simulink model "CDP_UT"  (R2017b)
settings: Solver=FixedStepDiscrete  StartTime=0.0  StopTime=10.0  FixedStep=0.01  RelTol=1e-3  EnableMultiTasking=on
undefined symbols (not defined in the file): ASWTYPE_FALSE, ASWTYPE_TRUE, CaCDP_CellTempNTCVoltTable_mV, CaCDP_CellTempTable_C, CaCDP_CMUPCBTempNTCVoltTable_mV, CaCDP_CMUPCBTempTable_C, CbCDP_DiffBusbarTempStateCheck_flg, CbCDP_DiffCellTempStateCheck_flg, CbCDP_DiffCellVoltStateCheck_flg, CbCDP_IgnorUpdateVld_flg, CbCDP_MaxBusbarTempStateCheck_flg, CbCDP_MaxCellTempStateCheck_flg, CbCDP_MaxCellVoltStateCheck_flg, CbCDP_MinBusbarTempStateCheck_flg, CbCDP_MinCellTempStateCheck_flg, CbCDP_MinCellVoltStateCheck_flg, CcCDP_AFETempConfig_numb, CcCDP_AFETempFltThd_C, CcCDP_AFETempFltThdHys_C, CcCDP_BusbarTempRngFltHiThrd_C, CcCDP_BusbarTempRngFltLowThrd_C, CcCDP_CellDiffFltLevel1_mV, CcCDP_CellDiffFltLevel2_mV, CcCDP_CellDiffFltLevel3_mV, CcCDP_CellTempLowerLimit_C, CcCDP_CellTempRngFltHiThrd_C, CcCDP_CellTempRngFltLowThrd_C, CcCDP_CellTempUpperLimit_C, CcCDP_CellVoltConfig_numb, CcCDP_CellVoltLowerLimit_mV, CcCDP_CellVoltRngHiThrd_mV, CcCDP_CellVoltRngLowThrd_mV, CcCDP_CellVoltUpdateThrd_numb, CcCDP_CellVoltUpperLimit_mV, CcCDP_ChrgMaxCellTempFltLv1Thrd_C, CcCDP_ChrgMaxCellTempFltLv2Thrd_C, CcCDP_ChrgMaxCellTempFltLv3Thrd_C, CcCDP_ChrgMaxCellTempReturnDiff_C, CcCDP_ChrgMinCellTempFltLv1Thrd_C, CcCDP_ChrgMinCellTempFltLv2Thrd_C, CcCDP_ChrgMinCellTempFltLv3Thrd_C, CcCDP_ChrgMinCellTempReturnDiff_C, CcCDP_CMUPCBTempConfig_numb, CcCDP_CMUPCBTempFltThd_C, CcCDP_CMUPCBTempFltThdHys_C, CcCDP_DiffBusbarTempFltLevel1Thrd_C, CcCDP_DiffBusbarTempFltLevel2Thrd_C, CcCDP_DiffBusbarTempReturnDifference_C, CcCDP_DiffCellTempFltLevel1Thrd_C, CcCDP_DiffCellTempFltLevel2Thrd_C, CcCDP_DiffCellTempReturnDifference_C, CcCDP_DiffCellVoltReturnDifference_mV, CcCDP_DiffVoltCheckMaxCellTempCondition_C, CcCDP_DiffVoltCheckMaxCellVoltCondition_mV, CcCDP_DiffVoltCheckMinCellTempCondition_C, CcCDP_DiffVoltCheckMinCellVoltCondition_mV, CcCDP_DiffVoltCheckPackCurrCondition_A, CcCDP_MaxAFETempIniVal_C, CcCDP_MaxBusbarTempFltLevel1Thrd_C, CcCDP_MaxBusbarTempFltLevel2Thrd_C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
libraries: AIWAYS_Powertrain_BMS_lib x148, simulink x8
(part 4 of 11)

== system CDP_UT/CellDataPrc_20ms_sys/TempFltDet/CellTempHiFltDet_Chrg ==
  GbCDP_AllCellTempVld_flg : Inport
  GcCDP_MaxCellTemp_C : Inport  Port=2
  LbCDP_AnyCellTempVld_flg : Inport  Port=3
  LbCDP_ChrgWkUp_flg : Inport  Port=4
  ChrgCellTempHiFltDet_sys : Subsystem
  ChrgMaxTempCheck_Condition : Subsystem
  GbCDP_ChrgCellTempHiFltLv3_flg : Outport
  GbCDP_ChrgCellTempHiFltLv2_flg : Outport  Port=2
  GbCDP_ChrgCellTempHiFltLv1_flg : Outport  Port=3
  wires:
  LbCDP_ChrgWkUp_flg/1 -> ChrgMaxTempCheck_Condition/3(LbCDP_ChrgWkUp_flg)
  ChrgMaxTempCheck_Condition/1(LbCDP_ChrgMaxTempChkCond_flg) -> ChrgCellTempHiFltDet_sys/1(LbCDP_ChrgMaxTempChkCond_flg)
  LbCDP_AnyCellTempVld_flg/1 -> ChrgMaxTempCheck_Condition/2(LbCDP_AnyCellTempVld_flg)
  ChrgCellTempHiFltDet_sys/3(GbCDP_ChrgCellTempHiFltLv1_flg) -> GbCDP_ChrgCellTempHiFltLv1_flg/1
  ChrgCellTempHiFltDet_sys/2(GbCDP_ChrgCellTempHiFltLv2_flg) -> GbCDP_ChrgCellTempHiFltLv2_flg/1
  ChrgCellTempHiFltDet_sys/1(GbCDP_ChrgCellTempHiFltLv3_flg) -> GbCDP_ChrgCellTempHiFltLv3_flg/1
  GbCDP_AllCellTempVld_flg/1 -> ChrgMaxTempCheck_Condition/1(GbCDP_AllCellTempVld_flg)
  GcCDP_MaxCellTemp_C/1 -> ChrgCellTempHiFltDet_sys/2(GcCDP_MaxCellTemp_C)

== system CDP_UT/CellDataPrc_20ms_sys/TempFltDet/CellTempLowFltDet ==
  GbCDP_AllCellTempVld_flg : Inport
  GcCDP_MinCellTemp_C : Inport  Port=2
  LbCDP_AnyCellTempVld_flg : Inport  Port=3
  LbCDP_ChrgWkUp_flg : Inport  Port=4
  MinCellTemp_SateSwitch_Sys : Subsystem
  MinTempCheck_Condition : Subsystem
  GbCDP_CellTempLowFltLv3_flg : Outport
  GbCDP_CellTempLowFltLv2_flg : Outport  Port=2
  GbCDP_CellTempLowFltLv1_flg : Outport  Port=3
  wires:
  GcCDP_MinCellTemp_C/1 -> MinCellTemp_SateSwitch_Sys/2(GcCDP_MinCellTemp_C)
  GbCDP_AllCellTempVld_flg/1 -> MinTempCheck_Condition/1(GbCDP_AllCellTempVld_flg)
  MinCellTemp_SateSwitch_Sys/1(GbCDP_CellTempLowFltLv3_flg) -> GbCDP_CellTempLowFltLv3_flg/1
  MinCellTemp_SateSwitch_Sys/2(GbCDP_CellTempLowFltLv2_flg) -> GbCDP_CellTempLowFltLv2_flg/1
  MinCellTemp_SateSwitch_Sys/3(GbCDP_CellTempLowFltLv1_flg) -> GbCDP_CellTempLowFltLv1_flg/1
  LbCDP_AnyCellTempVld_flg/1 -> MinTempCheck_Condition/2(LbCDP_AnyCellTempVld_flg)
  MinTempCheck_Condition/1(LbCDP_MinTempCheckCondition_flg) -> MinCellTemp_SateSwitch_Sys/1(LbCDP_MinTempCheckCondition_flg)
  LbCDP_ChrgWkUp_flg/1 -> MinTempCheck_Condition/3(LbCDP_ChrgWkUp_flg)

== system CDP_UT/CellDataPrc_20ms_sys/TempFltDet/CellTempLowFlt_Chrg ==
  GbCDP_AllCellTempVld_flg : Inport
  GcCDP_MinCellTemp_C : Inport  Port=2
  LbCDP_AnyCellTempVld_flg : Inport  Port=3
  LbCDP_ChrgWkUp_flg : Inport  Port=4
  ChrgMinCellTemp_SateSwitch_Sys : Subsystem
  ChrgMinTempCheck_Condition : Subsystem
  GbCDP_ChrgCellTempLowFltLv3_flg : Outport
  GbCDP_ChrgCellTempLowFltLv2_flg : Outport  Port=2
  GbCDP_ChrgCellTempLowFltLv1_flg : Outport  Port=3
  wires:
  LbCDP_ChrgWkUp_flg/1 -> ChrgMinTempCheck_Condition/3(LbCDP_ChrgWkUp_flg)
  ChrgMinTempCheck_Condition/1(LbCDP_ChrgMinTempChkCond_flg) -> ChrgMinCellTemp_SateSwitch_Sys/1(LbCDP_ChrgMinTempChkCond_flg)
  LbCDP_AnyCellTempVld_flg/1 -> ChrgMinTempCheck_Condition/2(LbCDP_AnyCellTempVld_flg)
  ChrgMinCellTemp_SateSwitch_Sys/3(GbCDP_ChrgCellTempLowFltLv1_flg) -> GbCDP_ChrgCellTempLowFltLv1_flg/1
  ChrgMinCellTemp_SateSwitch_Sys/2(GbCDP_ChrgCellTempLowFltLv2_flg) -> GbCDP_ChrgCellTempLowFltLv2_flg/1
  ChrgMinCellTemp_SateSwitch_Sys/1(GbCDP_ChrgCellTempLowFltLv3_flg) -> GbCDP_ChrgCellTempLowFltLv3_flg/1
  GbCDP_AllCellTempVld_flg/1 -> ChrgMinTempCheck_Condition/1(GbCDP_AllCellTempVld_flg)
  GcCDP_MinCellTemp_C/1 -> ChrgMinCellTemp_SateSwitch_Sys/2(GcCDP_MinCellTemp_C)

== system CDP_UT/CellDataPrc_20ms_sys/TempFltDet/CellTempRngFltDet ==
  GcCDP_MaxCellTemp_C : Inport
  GcCDP_MinCellTemp_C : Inport  Port=2
  LbCDP_AnyCellTempVld_flg : Inport  Port=3
  CellTempRngHiFltDet_sys : Subsystem
  CellTempRngLowFltDet_sys : Subsystem
  TempRngHiCheck_Condition : Subsystem
  TempRngLowCheck_Condition : Subsystem
  GbCDP_CellTempRngHiFlt_flg : Outport
  GbCDP_CellTempRngLowFlt_flg : Outport  Port=2
  LbCDP_CellTempRngHiFlt_flg : Outport  Port=3
  LbCDP_CellTempRngLowFlt_flg : Outport  Port=4
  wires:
  GcCDP_MaxCellTemp_C/1 -> CellTempRngHiFltDet_sys/2(GcCDP_MaxCellTemp_C)
  LbCDP_AnyCellTempVld_flg/1 -> TempRngLowCheck_Condition/1(LbCDP_AnyCellTempVld_flg), TempRngHiCheck_Condition/1(LbCDP_AnyCellTempVld_flg)
  CellTempRngHiFltDet_sys/1(LbCDP_CellTempRngHiFlt_flg) -> LbCDP_CellTempRngHiFlt_flg/1
  CellTempRngHiFltDet_sys/2(GbCDP_CellTempRngHiFlt_flg) -> GbCDP_CellTempRngHiFlt_flg/1
  GcCDP_MinCellTemp_C/1 -> CellTempRngLowFltDet_sys/2(GcCDP_MinCellTemp_C)
  TempRngLowCheck_Condition/1(LbCDP_CellTempRngLowChk_flg) -> CellTempRngLowFltDet_sys/1(LbCDP_CellTempRngLowChk_flg)
  CellTempRngLowFltDet_sys/1(LbCDP_CellTempRngLowFlt_flg) -> LbCDP_CellTempRngLowFlt_flg/1
  CellTempRngLowFltDet_sys/2(GbCDP_CellTempRngLowFlt_flg) -> GbCDP_CellTempRngLowFlt_flg/1
  TempRngHiCheck_Condition/1(LbCDP_CellTempRngHiChk_flg) -> CellTempRngHiFltDet_sys/1(LbCDP_CellTempRngHiChk_flg)

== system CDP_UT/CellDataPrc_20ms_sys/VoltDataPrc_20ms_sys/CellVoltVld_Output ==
  GaISP_CellVoltVld_numb : Inport
  GeISP_CmuReIninSts_enum : Inport  Port=2
  Bitwise Logical Operator : simulink/Logic and Bit Operations/Bitwise Operator  logicop=AND  UseBitMask=on  BitMask=CDP_CONST97_NUMB  BitMaskRealWorld=Stored Integer
  Constant1 : Constant  Value=Enum_ISPCmuReIninSts.Enum_ISPCmuReIninSts_InintProcess
  Constant2 : Constant  Value=CDP_CONST0_NUMB
  Data Type Conversion : DataTypeConversion
  Logical Operator2 : Logic  Operator=OR  AllPortsSameDT=off  OutDataTypeStr=boolean
  OverWrite5 : AIWAYS_Powertrain_BMS_lib/Signals/OverWrite  OverWrite_Value=CaCDP_CellVoltVldOvr_flg  OverWrite_flag=CbCDP_CellVoltVldOvrSwt_flg
  Relational Operator1 : RelationalOperator  Operator===  OutDataTypeStr=boolean
  Relational Operator2 : RelationalOperator  Operator===  OutDataTypeStr=boolean
  LaCDP_CellVoltVld_flg : Outport
  GaCDP_CellVoltVld_flg : Outport  Port=2
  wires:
  OverWrite5/1 -> GaCDP_CellVoltVld_flg/1  "GaCDP_CellVoltVld_flg"
  GeISP_CmuReIninSts_enum/1 -> Data Type Conversion/1
  Logical Operator2/1 -> LaCDP_CellVoltVld_flg/1, OverWrite5/1  "LaCDP_CellVoltVld_flg"
  Relational Operator1/1 -> Logical Operator2/2
  Constant1/1 -> Relational Operator1/2
  Data Type Conversion/1 -> Relational Operator1/1
  Relational Operator2/1 -> Logical Operator2/1
  Constant2/1 -> Relational Operator2/2
  GaISP_CellVoltVld_numb/1 -> Bitwise Logical Operator/1
  Bitwise Logical Operator/1 -> Relational Operator2/1

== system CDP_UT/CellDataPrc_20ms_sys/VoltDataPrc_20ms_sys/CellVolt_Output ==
  GaISP_CellVolt_mV : Inport
  GaISP_CellVoltVld_numb : Inport  Port=2
  GeISP_CmuReIninSts_enum : Inport  Port=3
  GaISP_CellVoltUpdCnt_numb : Inport  Port=4
  GeUDS_CapSel_enum : Inport  Port=5
  GcUDS_CellVoltNum_numb : Inport  Port=6
  Bitwise Logical Operator : simulink/Logic and Bit Operations/Bitwise Operator  logicop=AND  UseBitMask=on  BitMask=CDP_CONST97_NUMB  BitMaskRealWorld=Stored Integer
  CellVolt_SignalFilt : Subsystem
  Comparison1 : RelationalOperator  Operator===  OutDataTypeStr=boolean
  Comparison4 : RelationalOperator  Operator===  OutDataTypeStr=boolean
  Constant1 : Constant  Value=Enum_ISPCmuReIninSts.Enum_ISPCmuReIninSts_InintProcess
  Constant2 : Constant  Value=CDP_CONST0_NUMB
  Constant3 : Constant  Value=CDP_CONST0_NUMB
  Constant4 : Constant  Value=CbCDP_IgnorUpdateVld_flg
  Constant5 : Constant  Value=ASWTYPE_FALSE
  Data Type Conversion : DataTypeConversion
  Logical Operator1 : Logic  Operator=OR  AllPortsSameDT=off  OutDataTypeStr=boolean
  Logical Operator2 : Logic  Operator=OR  AllPortsSameDT=off  OutDataTypeStr=boolean
  Relational Operator : RelationalOperator  Operator=~=  OutDataTypeStr=boolean
  Relational Operator1 : RelationalOperator  Operator===  OutDataTypeStr=boolean
  Switch : Switch  Criteria=u2 ~= 0
  Switch1 : Switch  Criteria=u2 ~= 0  Threshold=1  RndMeth=Zero
  Unit Delay : UnitDelay  SampleTime=-1  StateName=StateName
  LaCDP_CellVolt_mV : Outport
  GaCDP_CellVolt_mV : Outport  Port=2
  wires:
  Data Type Conversion/1 -> Relational Operator1/1
  Switch/1 -> CellVolt_SignalFilt/1(LaCDP_CellVolt_mV), LaCDP_CellVolt_mV/1, Unit Delay/1  "LaCDP_CellVolt_mV"
  Constant1/1 -> Relational Operator1/2
  Relational Operator1/1 -> Logical Operator2/2
  GaISP_CellVoltVld_numb/1 -> Bitwise Logical Operator/1
  GaISP_CellVolt_mV/1 -> Switch/3
  Logical Operator2/1 -> CellVolt_SignalFilt/2(LaCDP_CellVoltUpdateVld_flg), Switch/2
  Unit Delay/1 -> Switch/1
  GeISP_CmuReIninSts_enum/1 -> Data Type Conversion/1
  Constant2/1 -> Relational Operator/2
  Bitwise Logical Operator/1 -> Relational Operator/1
  Relational Operator/1 -> Logical Operator1/1, Switch1/1
  GaISP_CellVoltUpdCnt_numb/1 -> Comparison4/1
  Constant4/1 -> Switch1/2
  Constant3/1 -> Comparison4/2
  Logical Operator1/1 -> Switch1/3
  Comparison4/1 -> Comparison1/1
  Switch1/1 -> Logical Operator2/1
  Constant5/1 -> Comparison1/2
  Comparison1/1 -> Logical Operator1/2
  GeUDS_CapSel_enum/1 -> CellVolt_SignalFilt/3(GeUDS_CapSel_enum)
  CellVolt_SignalFilt/1(GaCDP_CellVolt_mV) -> GaCDP_CellVolt_mV/1
  GcUDS_CellVoltNum_numb/1 -> CellVolt_SignalFilt/4(GcUDS_CellVoltNum_numb)

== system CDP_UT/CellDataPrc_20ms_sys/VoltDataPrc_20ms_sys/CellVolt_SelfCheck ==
  GeMSM_BMUState_enum : Inport
  GbCDP_SumCellVoltVld_flg : Inport  Port=2
  GcCDP_MaxCellVolt_mV : Inport  Port=3
  GcCDP_MinCellVolt_mV : Inport  Port=4
  Constant : Constant  Value=Enum_MSMBMUState.Enum_MSMBMUState_Standby
  Constant1 : Constant  Value=ASWTYPE_TRUE
  Constant2 : Constant  Value=CcCDP_CellVoltLowerLimit_mV
  Constant3 : Constant  Value=CcCDP_CellVoltUpperLimit_mV
  Data Type Conversion1 : DataTypeConversion
  Logical Operator : Logic  Inputs=4  AllPortsSameDT=off  OutDataTypeStr=boolean
  OverWrite : AIWAYS_Powertrain_BMS_lib/Signals/OverWrite  OverWrite_Value=CbCDP_CellVoltSelfChckOvr_flg  OverWrite_flag=CbCDP_CellVoltSelfChckOvrSwt_flg
  Relational Operator : RelationalOperator  Operator===  OutDataTypeStr=boolean
  Relational Operator1 : RelationalOperator  OutDataTypeStr=boolean
  Relational Operator2 : RelationalOperator  Operator=<=  OutDataTypeStr=boolean
  Relational Operator4 : RelationalOperator  Operator===  OutDataTypeStr=boolean
  GbCDP_CellVoltSelfChck_flg : Outport
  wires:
  GeMSM_BMUState_enum/1 -> Data Type Conversion1/1
  Constant/1 -> Relational Operator4/2
  Relational Operator1/1 -> Logical Operator/3
  Relational Operator2/1 -> Logical Operator/2
  Logical Operator/1 -> OverWrite/1
  GcCDP_MinCellVolt_mV/1 -> Relational Operator1/1
  Constant2/1 -> Relational Operator1/2
  GbCDP_SumCellVoltVld_flg/1 -> Relational Operator/1
  Constant1/1 -> Relational Operator/2
  Relational Operator/1 -> Logical Operator/1
  OverWrite/1 -> GbCDP_CellVoltSelfChck_flg/1  "GbCDP_CellVoltSelfChck_flg"
  GcCDP_MaxCellVolt_mV/1 -> Relational Operator2/1
  Constant3/1 -> Relational Operator2/2
  Relational Operator4/1 -> Logical Operator/4
  Data Type Conversion1/1 -> Relational Operator4/1

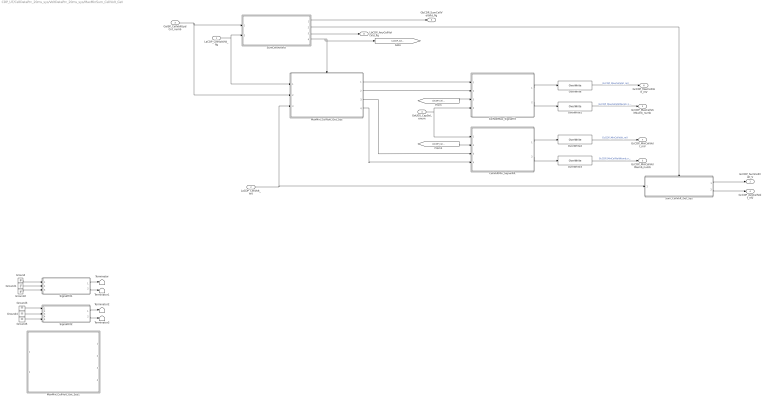
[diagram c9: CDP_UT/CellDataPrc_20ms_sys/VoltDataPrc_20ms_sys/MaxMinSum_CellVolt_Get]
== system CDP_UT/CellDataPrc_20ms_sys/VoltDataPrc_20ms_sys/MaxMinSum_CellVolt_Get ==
  LaCDP_CellVoltVld_flg : Inport
  LaCDP_CellVolt_mV : Inport  Port=2
  GaISP_CellVoltUpdCnt_numb : Inport  Port=3
  GeUDS_CapSel_enum : Inport  Port=4
  CellVoltMax_SignalFilt : Subsystem
  CellVoltMin_SignalFilt : Subsystem
  Ground{,1..5} (6 alike) : Ground
  MaxMin_CellVolt_Get_Sys : Subsystem
  MaxMin_CellVolt_Get_Sys1 : Subsystem  Commented=on
  OverWrite : AIWAYS_Powertrain_BMS_lib/Signals/OverWrite  OverWrite_Value=CcCDP_MaxCellVoltOvr_mV  OverWrite_flag=CbCDP_MaxCellVoltOvrSwt_flg
  OverWrite1 : AIWAYS_Powertrain_BMS_lib/Signals/OverWrite  OverWrite_Value=CcCDP_MaxCellVoltNumbOvr_numb  OverWrite_flag=CbCDP_MaxCellVoltNumbOvrSwt_flg
  OverWrite2 : AIWAYS_Powertrain_BMS_lib/Signals/OverWrite  OverWrite_Value=CcCDP_MinCellVoltOvr_mV  OverWrite_flag=CbCDP_MinCellVoltOvrSwt_flg
  OverWrite3 : AIWAYS_Powertrain_BMS_lib/Signals/OverWrite  OverWrite_Value=CcCDP_MinCellVoltNumbOvr_numb  OverWrite_flag=CbCDP_MinCellVoltNumbOvrSwt_flg
  SignalFilt1 : Subsystem  Commented=on
  SignalFilt2 : Subsystem  Commented=on
  SumCellVoltVld : Subsystem
  Sum_CellVolt_Get_Sys : Subsystem
  Terminator{,1..3} (4 alike) : Terminator
  GcCDP_SumCellVolt_V : Outport
  GcCDP_MaxCellVoltNumb_numb : Outport  Port=2
  GcCDP_MinCellVoltNumb_numb : Outport  Port=3
  GcCDP_AvgCellVolt_mV : Outport  Port=4
  GbCDP_SumCellVoltVld_flg : Outport  Port=5
  GcCDP_MaxCellVolt_mV : Outport  Port=6
  GcCDP_MinCellVolt_mV : Outport  Port=7
  LbCDP_AnyCellVoltVld_flg : Outport  Port=8
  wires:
  SumCellVoltVld/1(GbCDP_SumCellVoltVld_flg) -> GbCDP_SumCellVoltVld_flg/1
  LaCDP_CellVoltVld_flg/1 -> SumCellVoltVld/2(LaCDP_CellVoltVld_flg), MaxMin_CellVolt_Get_Sys/1(LaCDP_CellVoltVld_flg)
  LaCDP_CellVolt_mV/1 -> Sum_CellVolt_Get_Sys/1(LaCDP_CellVolt_mV), MaxMin_CellVolt_Get_Sys/3(LaCDP_CellVolt_mV)
  Sum_CellVolt_Get_Sys/1(GcCDP_SumCellVolt_V) -> GcCDP_SumCellVolt_V/1
  Sum_CellVolt_Get_Sys/2(GcCDP_AvgCellVolt_mV) -> GcCDP_AvgCellVolt_mV/1
  SumCellVoltVld/3(LbCDP_AnyCellVoltVld_flg) -> LbCDP_AnyCellVoltVld_flg/1
  SumCellVoltVld/2(LbCDP_SumCellVoltVld_flg) -> Sum_CellVolt_Get_Sys/Enable
  SignalFilt1/1(Output_Value) -> Terminator/1
  SignalFilt1/2(Output_Numb) -> Terminator1/1
  Ground/1 -> SignalFilt1/1(Input_Value)
  Ground1/1 -> SignalFilt1/2(Input_Numb)
  Ground2/1 -> SignalFilt1/3(GeUDS_CapSel_enum)
  Ground5/1 -> SignalFilt2/5(InputValueUpdate)
  Ground4/1 -> SignalFilt2/3(GeUDS_CapSel_enum)
  Ground3/1 -> SignalFilt2/1(Input_Value)
  SignalFilt2/2(Output_Numb) -> Terminator3/1
  SignalFilt2/1(Output_Value) -> Terminator2/1
  MaxMin_CellVolt_Get_Sys/1(LcCDP_MaxCellVolt_mV) -> CellVoltMax_SignalFilt/1(LcCDP_MaxCellVolt_mV)
  MaxMin_CellVolt_Get_Sys/2(LcCDP_MaxCellVoltNumb_numb) -> CellVoltMax_SignalFilt/2(LcCDP_MaxCellVoltNumb_numb)
  GaISP_CellVoltUpdCnt_numb/1 -> MaxMin_CellVolt_Get_Sys/2(GaISP_CellVoltUpdCnt_numb), SumCellVoltVld/1(GaISP_CellVoltUpdCnt_numb)
  CellVoltMax_SignalFilt/1(GcCDP_MaxCellVolt_mV) -> OverWrite/1
  OverWrite/1 -> GcCDP_MaxCellVolt_mV/1  "GcCDP_MaxCellVolt_mV"
  CellVoltMax_SignalFilt/2(GcCDP_MaxCellVoltNumb_numb) -> OverWrite1/1
  OverWrite1/1 -> GcCDP_MaxCellVoltNumb_numb/1  "GcCDP_MaxCellVoltNumb_numb"
  MaxMin_CellVolt_Get_Sys/3(LcCDP_MinCellVolt_mV) -> CellVoltMin_SignalFilt/3(LcCDP_MinCellVolt_mV)
  MaxMin_CellVolt_Get_Sys/4(LcCDP_MinCellVoltNumb_numb) -> CellVoltMin_SignalFilt/4(LcCDP_MinCellVoltNumb_numb)
  OverWrite2/1 -> GcCDP_MinCellVolt_mV/1  "GcCDP_MinCellVolt_mV"
  CellVoltMin_SignalFilt/1(GcCDP_MinCellVolt_mV) -> OverWrite2/1
  CellVoltMin_SignalFilt/2(GcCDP_MinCellVoltNumb_numb) -> OverWrite3/1
  OverWrite3/1 -> GcCDP_MinCellVoltNumb_numb/1  "GcCDP_MinCellVoltNumb_numb"
  SumCellVoltVld/4(LbCDP_CellVoltUpdateVld_flg) -> MaxMin_CellVolt_Get_Sys/Enable, [LbCDP_CellVoltUpdateVld_flg]
  GeUDS_CapSel_enum/1 -> CellVoltMin_SignalFilt/1(GeUDS_CapSel_enum), CellVoltMax_SignalFilt/4(GeUDS_CapSel_enum)
  [LbCDP_CellVoltUpdateVld_flg] -> CellVoltMax_SignalFilt/3(LbCDP_CellVoltUpdateVld_flg)
  [LbCDP_CellVoltUpdateVld_flg] -> CellVoltMin_SignalFilt/2(LbCDP_CellVoltUpdateVld_flg)

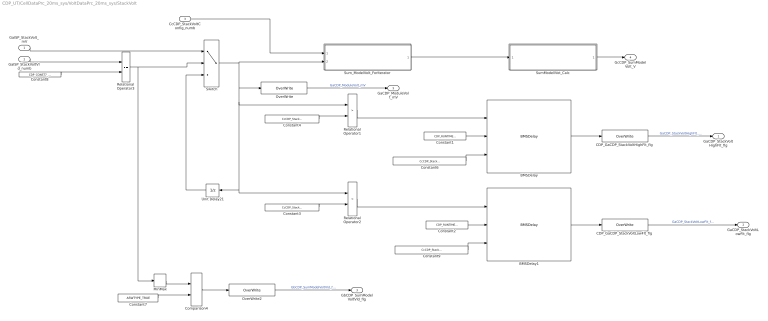
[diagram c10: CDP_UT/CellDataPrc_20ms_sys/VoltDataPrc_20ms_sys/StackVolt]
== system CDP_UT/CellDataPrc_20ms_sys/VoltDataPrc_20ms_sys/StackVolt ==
  GaISP_StackVolt_mV : Inport
  GaISP_StackVoltVld_numb : Inport  Port=2
  CcCDP_StackVoltConfig_numb : Inport  Port=3
  BMSDelay : AIWAYS_Powertrain_BMS_lib/Debounce & Delay/BMSDelay
  BMSDelay1 : AIWAYS_Powertrain_BMS_lib/Debounce & Delay/BMSDelay
  CDP_GaCDP_StackVoltHighFlt_flg : AIWAYS_Powertrain_BMS_lib/Signals/OverWrite  OverWrite_Value=CaCDP_StackVoltHighFltOvr_flg  OverWrite_flag=CbCDP_StackVoltHighFltOvrSwt_flg
  CDP_GaCDP_StackVoltLowFlt_flg : AIWAYS_Powertrain_BMS_lib/Signals/OverWrite  OverWrite_Value=CaCDP_StackVoltLowFltOvr_flg  OverWrite_flag=CbCDP_StackVoltLowFltOvrSwt_flg
  Comparison4 : RelationalOperator  Operator===  OutDataTypeStr=boolean
  Constant1 : Constant  Value=CDP_RUNTIME20_MS
  Constant2 : Constant  Value=CDP_RUNTIME20_MS
  Constant3 : Constant  Value=CcCDP_StackVoltLow_mV
  Constant4 : Constant  Value=CcCDP_StackVoltHigh_mV
  Constant6 : Constant  Value=CcCDP_StackVoltHighDelayTi_ms
  Constant7 : Constant  Value=ASWTYPE_TRUE
  Constant8 : Constant  Value=CDP_CONST7_NUMB
  Constant9 : Constant  Value=CcCDP_StackVoltLowDelayTi_ms
  MinMax : MinMax  OutDataTypeStr=Inherit: Inherit via back propagation  RndMeth=Zero
  OverWrite : AIWAYS_Powertrain_BMS_lib/Signals/OverWrite  OverWrite_Value=CaCDP_ModuleVoltOvr_mV  OverWrite_flag=CbCDP_ModuleVoltOvrSwt_flg
  OverWrite2 : AIWAYS_Powertrain_BMS_lib/Signals/OverWrite  OverWrite_Value=CbCDP_SumModelVoltVldOvr_flg  OverWrite_flag=CbCDP_SumModelVoltVldOvrSwt_flg
  Relational Operator1 : RelationalOperator  Operator=>  OutDataTypeStr=boolean
  Relational Operator2 : RelationalOperator  Operator=<  OutDataTypeStr=boolean
  Relational Operator3 : RelationalOperator  Operator===  OutDataTypeStr=boolean
  SumModellVot_Calc : Subsystem
  Sum_ModelVolt_ForIterator : Subsystem
  Switch : Switch  Criteria=u2 ~= 0  Threshold=1  RndMeth=Zero
  Unit Delay21 : UnitDelay  SampleTime=-1  StateName=StateName
  GaCDP_StackVoltHighFlt_flg : Outport
  GaCDP_StackVoltLowFlt_flg : Outport  Port=2
  GbCDP_SumModelVoltVld_flg : Outport  Port=3
  GcCDP_SumModelVolt_V : Outport  Port=4
  GaCDP_ModuleVolt_mV : Outport  Port=5
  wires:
  BMSDelay1/1 -> CDP_GaCDP_StackVoltLowFlt_flg/1
  CDP_GaCDP_StackVoltHighFlt_flg/1 -> GaCDP_StackVoltHighFlt_flg/1  "GaCDP_StackVoltHighFlt_flg"
  GaISP_StackVolt_mV/1 -> Switch/1
  CDP_GaCDP_StackVoltLowFlt_flg/1 -> GaCDP_StackVoltLowFlt_flg/1  "GaCDP_StackVoltLowFlt_flg"
  BMSDelay/1 -> CDP_GaCDP_StackVoltHighFlt_flg/1
  Relational Operator3/1 -> MinMax/1, Switch/2
  Unit Delay21/1 -> Switch/3
  Constant9/1 -> BMSDelay1/3
  Constant8/1 -> Relational Operator3/2
  Constant6/1 -> BMSDelay/3
  Relational Operator2/1 -> BMSDelay1/1
  Constant4/1 -> Relational Operator1/2
  Constant1/1 -> BMSDelay/2
  Relational Operator1/1 -> BMSDelay/1
  Constant3/1 -> Relational Operator2/2
  Constant2/1 -> BMSDelay1/2
  MinMax/1 -> Comparison4/1
  OverWrite2/1 -> GbCDP_SumModelVoltVld_flg/1  "GbCDP_SumModelVoltVld_flg"
  Constant7/1 -> Comparison4/2
  SumModellVot_Calc/1(GcCDP_SumModelVolt_V) -> GcCDP_SumModelVolt_V/1
  Comparison4/1 -> OverWrite2/1
  CcCDP_StackVoltConfig_numb/1 -> Sum_ModelVolt_ForIterator/1(CcCDP_StackVoltConfig_numb)
  Sum_ModelVolt_ForIterator/1(LcCDP_SumModelVolt_mV) -> SumModellVot_Calc/1(LcCDP_SumModelVolt_mV)
  GaISP_StackVoltVld_numb/1 -> Relational Operator3/1
  OverWrite/1 -> GaCDP_ModuleVolt_mV/1  "GaCDP_ModuleVolt_mV"
  Switch/1 -> OverWrite/1, Relational Operator2/1, Unit Delay21/1, Relational Operator1/1, Sum_ModelVolt_ForIterator/2(GaISP_StackVolt_mV)

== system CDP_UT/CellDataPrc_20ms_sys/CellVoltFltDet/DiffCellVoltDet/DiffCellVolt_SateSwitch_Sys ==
  LbCDP_DiffvoltCheckCondition_flg : Inport
  GcCDP_MaxCellVolt_mV : Inport  Port=2
  GcCDP_MinCellVolt_mV : Inport  Port=3
  LbCDP_CellVoltRngLowFlt_flg : Inport  Port=4
  LbCDP_CellVoltRngHiFlt_flg : Inport  Port=5
  Add : Sum  Inputs=+-
  Bus Creator : BusCreator  Inputs=4
  Bus Selector : BusSelector  OutputSignals=LcCDP_DiffCellVolt_mV,LbCDP_DiffvoltCheckCondition_flg,LbCDP_CellVoltRngLowFlt_flg,LbCDP_CellVoltRngHiFlt_flg
  Bus Selector1 : BusSelector  OutputSignals=LcCDP_DiffCellVolt_mV,LbCDP_DiffvoltCheckCondition_flg,LbCDP_CellVoltRngLowFlt_flg,LbCDP_CellVoltRngHiFlt_flg
  Bus Selector2 : BusSelector  OutputSignals=LcCDP_DiffCellVolt_mV,LbCDP_DiffvoltCheckCondition_flg,LbCDP_CellVoltRngLowFlt_flg,LbCDP_CellVoltRngHiFlt_flg
  CellVoltDiffFltLv1Det : Subsystem
  CellVoltDiffFltLv2Det : Subsystem
  CellVoltDiffFltLv3Det : Subsystem
  GbCDP_CellVoltDiffFltLv3_flg : Outport
  GbCDP_CellVoltDiffFltLv2_flg : Outport  Port=2
  GbCDP_CellVoltDiffFltLv1_flg : Outport  Port=3
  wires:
  Bus Creator/1 -> Bus Selector2/1, Bus Selector1/1, Bus Selector/1
  Add/1 -> Bus Creator/1  "LcCDP_DiffCellVolt_mV"
  GcCDP_MinCellVolt_mV/1 -> Add/2
  GcCDP_MaxCellVolt_mV/1 -> Add/1
  CellVoltDiffFltLv3Det/1(GbCDP_CellVoltDiffFltLv3_flg) -> GbCDP_CellVoltDiffFltLv3_flg/1
  CellVoltDiffFltLv2Det/1(GbCDP_CellVoltDiffFltLv2_flg) -> GbCDP_CellVoltDiffFltLv2_flg/1
  CellVoltDiffFltLv1Det/1(GbCDP_CellVoltDiffFltLv1_flg) -> GbCDP_CellVoltDiffFltLv1_flg/1
  LbCDP_DiffvoltCheckCondition_flg/1 -> Bus Creator/2
  Bus Selector/1 -> CellVoltDiffFltLv3Det/1(LcCDP_DiffCellVolt_mV)  "<LcCDP_DiffCellVolt_mV>"
  Bus Selector/2 -> CellVoltDiffFltLv3Det/2(LbCDP_DiffvoltCheckCondition_flg)  "<LbCDP_DiffvoltCheckCondition_flg>"
  LbCDP_CellVoltRngLowFlt_flg/1 -> Bus Creator/3
  LbCDP_CellVoltRngHiFlt_flg/1 -> Bus Creator/4
  Bus Selector/3 -> CellVoltDiffFltLv3Det/3(LbCDP_CellVoltRngLowFlt_flg)  "<LbCDP_CellVoltRngLowFlt_flg>"
  Bus Selector/4 -> CellVoltDiffFltLv3Det/4(LbCDP_CellVoltRngHiFlt_flg)  "<LbCDP_CellVoltRngHiFlt_flg>"
  Bus Selector1/1 -> CellVoltDiffFltLv2Det/1(LcCDP_DiffCellVolt_mV)  "<LcCDP_DiffCellVolt_mV>"
  Bus Selector1/2 -> CellVoltDiffFltLv2Det/2(LbCDP_DiffvoltCheckCondition_flg)  "<LbCDP_DiffvoltCheckCondition_flg>"
  Bus Selector1/3 -> CellVoltDiffFltLv2Det/3(LbCDP_CellVoltRngLowFlt_flg)  "<LbCDP_CellVoltRngLowFlt_flg>"
  Bus Selector1/4 -> CellVoltDiffFltLv2Det/4(LbCDP_CellVoltRngHiFlt_flg)  "<LbCDP_CellVoltRngHiFlt_flg>"
  Bus Selector2/1 -> CellVoltDiffFltLv1Det/1(LcCDP_DiffCellVolt_mV)  "<LcCDP_DiffCellVolt_mV>"
  Bus Selector2/2 -> CellVoltDiffFltLv1Det/2(LbCDP_DiffvoltCheckCondition_flg)  "<LbCDP_DiffvoltCheckCondition_flg>"
  Bus Selector2/3 -> CellVoltDiffFltLv1Det/3(LbCDP_CellVoltRngLowFlt_flg)  "<LbCDP_CellVoltRngLowFlt_flg>"
  Bus Selector2/4 -> CellVoltDiffFltLv1Det/4(LbCDP_CellVoltRngHiFlt_flg)  "<LbCDP_CellVoltRngHiFlt_flg>"

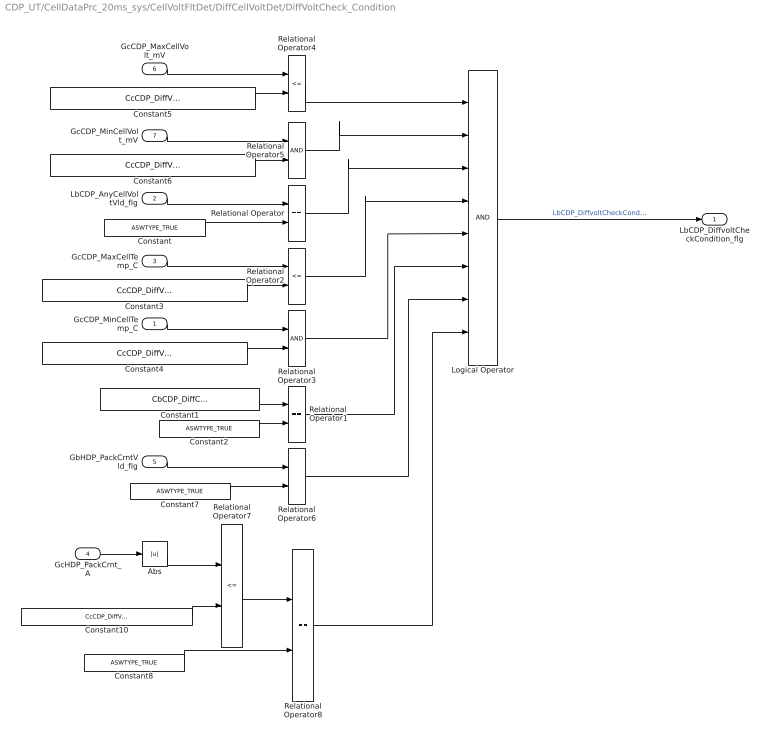
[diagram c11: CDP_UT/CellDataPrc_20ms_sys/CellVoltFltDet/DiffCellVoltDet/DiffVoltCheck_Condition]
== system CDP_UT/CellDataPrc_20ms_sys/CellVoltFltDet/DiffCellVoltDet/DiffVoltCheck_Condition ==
  GcCDP_MinCellTemp_C : Inport
  LbCDP_AnyCellVoltVld_flg : Inport  Port=2
  GcCDP_MaxCellTemp_C : Inport  Port=3
  GcHDP_PackCrnt_A : Inport  Port=4
  GbHDP_PackCrntVld_flg : Inport  Port=5
  GcCDP_MaxCellVolt_mV : Inport  Port=6
  GcCDP_MinCellVolt_mV : Inport  Port=7
  Abs : Abs
  Constant{,2,7..8} (4 alike) : Constant  Value=ASWTYPE_TRUE
  Constant1 : Constant  Value=CbCDP_DiffCellVoltStateCheck_flg
  Constant10 : Constant  Value=CcCDP_DiffVoltCheckPackCurrCondition_A
  Constant3 : Constant  Value=CcCDP_DiffVoltCheckMaxCellTempCondition_C
  Constant4 : Constant  Value=CcCDP_DiffVoltCheckMinCellTempCondition_C
  Constant5 : Constant  Value=CcCDP_DiffVoltCheckMaxCellVoltCondition_mV
  Constant6 : Constant  Value=CcCDP_DiffVoltCheckMinCellVoltCondition_mV
  Logical Operator : Logic  Inputs=8  AllPortsSameDT=off  OutDataTypeStr=boolean
  Relational Operator{,1,6,8} (4 alike) : RelationalOperator  Operator===  OutDataTypeStr=boolean
  Relational Operator2 : RelationalOperator  Operator=<=  OutDataTypeStr=boolean
  Relational Operator3 : RelationalOperator  OutDataTypeStr=boolean
  Relational Operator4 : RelationalOperator  Operator=<=  OutDataTypeStr=boolean
  Relational Operator5 : RelationalOperator  OutDataTypeStr=boolean
  Relational Operator7 : RelationalOperator  Operator=<=  OutDataTypeStr=boolean
  LbCDP_DiffvoltCheckCondition_flg : Outport
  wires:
  GcCDP_MinCellTemp_C/1 -> Relational Operator3/1
  Constant1/1 -> Relational Operator1/1
  Constant2/1 -> Relational Operator1/2
  Relational Operator8/1 -> Logical Operator/8
  Relational Operator3/1 -> Logical Operator/5
  Constant/1 -> Relational Operator/2
  Relational Operator7/1 -> Relational Operator8/1
  Logical Operator/1 -> LbCDP_DiffvoltCheckCondition_flg/1  "LbCDP_DiffvoltCheckCondition_flg"
  LbCDP_AnyCellVoltVld_flg/1 -> Relational Operator/1
  Constant6/1 -> Relational Operator5/2
  Constant3/1 -> Relational Operator2/2
  Relational Operator6/1 -> Logical Operator/7
  Relational Operator/1 -> Logical Operator/3
  Relational Operator2/1 -> Logical Operator/4
  Relational Operator5/1 -> Logical Operator/2
  GcCDP_MaxCellTemp_C/1 -> Relational Operator2/1
  Constant4/1 -> Relational Operator3/2
  Constant5/1 -> Relational Operator4/2
  Relational Operator1/1 -> Logical Operator/6
  GcCDP_MinCellVolt_mV/1 -> Relational Operator5/1
  GcCDP_MaxCellVolt_mV/1 -> Relational Operator4/1
  Constant7/1 -> Relational Operator6/2
  Relational Operator4/1 -> Logical Operator/1
  Constant10/1 -> Relational Operator7/2
  GcHDP_PackCrnt_A/1 -> Abs/1
  Constant8/1 -> Relational Operator8/2
  GbHDP_PackCrntVld_flg/1 -> Relational Operator6/1
  Abs/1 -> Relational Operator7/1

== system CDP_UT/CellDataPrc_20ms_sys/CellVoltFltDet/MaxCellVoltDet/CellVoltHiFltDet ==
  LbCDP_MaxVoltCheckCondition_flg : Inport
  GcCDP_MaxCellVolt_mV : Inport  Port=2
  LcCDP_CellHighFltLevel1_mV : Inport  Port=3
  LcCDP_CellHighFltLevel2_mV : Inport  Port=4
  LcCDP_CellHighFltLevel3_mV : Inport  Port=5
  GbCTC_ChrgHVMode_flg : Inport  Port=6
  Bus Creator : BusCreator  Inputs=6
  Bus Selector1 : BusSelector  OutputSignals=LbCDP_MaxVoltCheckCondition_flg,GcCDP_MaxCellVolt_mV,LcCDP_CellHighFltLevel2_mV,LcCDP_CellHighFltLevel3_mV
  Bus Selector2 : BusSelector  OutputSignals=LbCDP_MaxVoltCheckCondition_flg,GcCDP_MaxCellVolt_mV,LcCDP_CellHighFltLevel1_mV,LcCDP_CellHighFltLevel2_mV
  Bus Selector6 : BusSelector  OutputSignals=LbCDP_MaxVoltCheckCondition_flg,GcCDP_MaxCellVolt_mV,LcCDP_CellHighFltLevel3_mV
  CellVoltHiFltLv1Det : Subsystem
  CellVoltHiFltLv2Det : Subsystem
  CellVoltHiFltLv3Det : Subsystem
  GbCDP_CellVoltHiFltLv3_flg : Outport
  GbCDP_CellVoltHiFltLv2_flg : Outport  Port=2
  GbCDP_CellVoltHiFltLv1_flg : Outport  Port=3
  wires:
  Bus Creator/1 -> Bus Selector2/1, Bus Selector1/1, Bus Selector6/1
  CellVoltHiFltLv3Det/1(GbCDP_CellVoltHiFltLv3_flg) -> GbCDP_CellVoltHiFltLv3_flg/1
  CellVoltHiFltLv2Det/1(GbCDP_CellVoltHiFltLv2_flg) -> GbCDP_CellVoltHiFltLv2_flg/1
  CellVoltHiFltLv1Det/1(GbCDP_CellVoltHiFltLv1_flg) -> GbCDP_CellVoltHiFltLv1_flg/1
  GcCDP_MaxCellVolt_mV/1 -> Bus Creator/1
  LcCDP_CellHighFltLevel1_mV/1 -> Bus Creator/2
  LcCDP_CellHighFltLevel2_mV/1 -> Bus Creator/3
  LcCDP_CellHighFltLevel3_mV/1 -> Bus Creator/4
  GbCTC_ChrgHVMode_flg/1 -> Bus Creator/5
  Bus Selector1/1 -> CellVoltHiFltLv2Det/1(LbCDP_MaxVoltCheckCondition_flg)  "<LbCDP_MaxVoltCheckCondition_flg>"
  Bus Selector1/2 -> CellVoltHiFltLv2Det/2(GcCDP_MaxCellVolt_mV)  "<GcCDP_MaxCellVolt_mV>"
  Bus Selector1/3 -> CellVoltHiFltLv2Det/3(LcCDP_CellHighFltLevel2_mV)  "<LcCDP_CellHighFltLevel2_mV>"
  Bus Selector1/4 -> CellVoltHiFltLv2Det/4(LcCDP_CellHighFltLevel3_mV)  "<LcCDP_CellHighFltLevel3_mV>"
  Bus Selector2/1 -> CellVoltHiFltLv1Det/1(LbCDP_MaxVoltCheckCondition_flg)  "<LbCDP_MaxVoltCheckCondition_flg>"
  Bus Selector2/2 -> CellVoltHiFltLv1Det/2(GcCDP_MaxCellVolt_mV)  "<GcCDP_MaxCellVolt_mV>"
  Bus Selector2/3 -> CellVoltHiFltLv1Det/3(LcCDP_CellHighFltLevel1_mV)  "<LcCDP_CellHighFltLevel1_mV>"
  Bus Selector2/4 -> CellVoltHiFltLv1Det/4(LcCDP_CellHighFltLevel2_mV)  "<LcCDP_CellHighFltLevel2_mV>"
  Bus Selector6/1 -> CellVoltHiFltLv3Det/1(LbCDP_MaxVoltCheckCondition_flg)  "<LbCDP_MaxVoltCheckCondition_flg>"
  Bus Selector6/2 -> CellVoltHiFltLv3Det/2(GcCDP_MaxCellVolt_mV)  "<GcCDP_MaxCellVolt_mV>"
  Bus Selector6/3 -> CellVoltHiFltLv3Det/3(LcCDP_CellHighFltLevel3_mV)  "<LcCDP_CellHighFltLevel3_mV>"
  LbCDP_MaxVoltCheckCondition_flg/1 -> Bus Creator/6

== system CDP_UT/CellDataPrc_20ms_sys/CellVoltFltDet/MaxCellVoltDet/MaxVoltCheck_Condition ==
  GbCDP_SumCellVoltVld_flg : Inport
  GeMSM_BMUState_enum : Inport  Port=2
  LbCDP_AnyCellVoltVld_flg : Inport  Port=3
  Constant : Constant  Value=ASWTYPE_TRUE
  Constant1 : Constant  Value=CbCDP_MaxCellVoltStateCheck_flg
  Constant2 : Constant  Value=ASWTYPE_TRUE
  Constant3 : Constant  Value=Enum_MSMBMUState.Enum_MSMBMUState_Run
  Constant4 : Constant  Value=ASWTYPE_TRUE
  Data Type Conversion1 : DataTypeConversion
  Logical Operator : Logic  Inputs=3  AllPortsSameDT=off  OutDataTypeStr=boolean
  Relational Operator{,1..2,4} (4 alike) : RelationalOperator  Operator===  OutDataTypeStr=boolean
  Terminator : Terminator
  LbCDP_MaxVoltCheckCondition_flg : Outport
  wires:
  Logical Operator/1 -> LbCDP_MaxVoltCheckCondition_flg/1  "LbCDP_MaxVoltCheckCondition_flg"
  GbCDP_SumCellVoltVld_flg/1 -> Relational Operator/1
  Constant/1 -> Relational Operator/2
  Relational Operator/1 -> Terminator/1
  Constant2/1 -> Relational Operator1/2
  Constant1/1 -> Relational Operator1/1
  Relational Operator1/1 -> Logical Operator/2
  GeMSM_BMUState_enum/1 -> Data Type Conversion1/1
  Constant3/1 -> Relational Operator4/2
  Relational Operator4/1 -> Logical Operator/3
  Data Type Conversion1/1 -> Relational Operator4/1
  LbCDP_AnyCellVoltVld_flg/1 -> Relational Operator2/1
  Constant4/1 -> Relational Operator2/2
  Relational Operator2/1 -> Logical Operator/1

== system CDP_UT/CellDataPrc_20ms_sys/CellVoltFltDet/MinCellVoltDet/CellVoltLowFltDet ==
  LbCDP_MinVoltCheckCondition_flg : Inport
  GcCDP_MinCellVolt_mV : Inport  Port=2
  LcCDP_CellLowFltLevel1_mV : Inport  Port=3
  LcCDP_CellLowFltLevel2_mV : Inport  Port=4
  LcCDP_CellLowFltLevel3_mV : Inport  Port=5
  GbCTC_ChrgHVMode_flg : Inport  Port=6
  Bus Creator : BusCreator  Inputs=6
  Bus Selector : BusSelector  OutputSignals=LbCDP_MinVoltCheckCondition_flg,GcCDP_MinCellVolt_mV,LcCDP_CellLowFltLevel3_mV
  Bus Selector1 : BusSelector  OutputSignals=LbCDP_MinVoltCheckCondition_flg,GcCDP_MinCellVolt_mV,LcCDP_CellLowFltLevel2_mV,LcCDP_CellLowFltLevel3_mV
  Bus Selector2 : BusSelector  OutputSignals=LbCDP_MinVoltCheckCondition_flg,GcCDP_MinCellVolt_mV,LcCDP_CellLowFltLevel1_mV,LcCDP_CellLowFltLevel2_mV
  CellVoltLowFltLv1Det : Subsystem
  CellVoltLowFltLv2Det : Subsystem
  CellVoltLowFltLv3Det : Subsystem
  GbCDP_CellVoltLowFltLv3_flg : Outport
  GbCDP_CellVoltLowFltLv2_flg : Outport  Port=2
  GbCDP_CellVoltLowFltLv1_flg : Outport  Port=3
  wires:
  Bus Creator/1 -> Bus Selector2/1, Bus Selector1/1, Bus Selector/1
  GcCDP_MinCellVolt_mV/1 -> Bus Creator/1
  LcCDP_CellLowFltLevel1_mV/1 -> Bus Creator/2
  LcCDP_CellLowFltLevel2_mV/1 -> Bus Creator/3
  LcCDP_CellLowFltLevel3_mV/1 -> Bus Creator/4
  GbCTC_ChrgHVMode_flg/1 -> Bus Creator/5
  CellVoltLowFltLv3Det/1(GbCDP_CellVoltLowFltLv3_flg) -> GbCDP_CellVoltLowFltLv3_flg/1
  CellVoltLowFltLv2Det/1(GbCDP_CellVoltLowFltLv2_flg) -> GbCDP_CellVoltLowFltLv2_flg/1
  CellVoltLowFltLv1Det/1(GbCDP_CellVoltLowFltLv1_flg) -> GbCDP_CellVoltLowFltLv1_flg/1
  LbCDP_MinVoltCheckCondition_flg/1 -> Bus Creator/6
  Bus Selector1/1 -> CellVoltLowFltLv2Det/1(LbCDP_MinVoltCheckCondition_flg)  "<LbCDP_MinVoltCheckCondition_flg>"
  Bus Selector1/2 -> CellVoltLowFltLv2Det/2(GcCDP_MinCellVolt_mV)  "<GcCDP_MinCellVolt_mV>"
  Bus Selector1/3 -> CellVoltLowFltLv2Det/3(LcCDP_CellLowFltLevel2_mV)  "<LcCDP_CellLowFltLevel2_mV>"
  Bus Selector1/4 -> CellVoltLowFltLv2Det/4(LcCDP_CellLowFltLevel3_mV)  "<LcCDP_CellLowFltLevel3_mV>"
  Bus Selector2/1 -> CellVoltLowFltLv1Det/1(LbCDP_MinVoltCheckCondition_flg)  "<LbCDP_MinVoltCheckCondition_flg>"
  Bus Selector2/2 -> CellVoltLowFltLv1Det/2(GcCDP_MinCellVolt_mV)  "<GcCDP_MinCellVolt_mV>"
  Bus Selector2/3 -> CellVoltLowFltLv1Det/3(LcCDP_CellLowFltLevel1_mV)  "<LcCDP_CellLowFltLevel1_mV>"
  Bus Selector2/4 -> CellVoltLowFltLv1Det/4(LcCDP_CellLowFltLevel2_mV)  "<LcCDP_CellLowFltLevel2_mV>"
  Bus Selector/1 -> CellVoltLowFltLv3Det/1(LbCDP_MinVoltCheckCondition_flg)  "<LbCDP_MinVoltCheckCondition_flg>"
  Bus Selector/2 -> CellVoltLowFltLv3Det/2(GcCDP_MinCellVolt_mV)  "<GcCDP_MinCellVolt_mV>"
  Bus Selector/3 -> CellVoltLowFltLv3Det/3(LcCDP_CellLowFltLevel3_mV)  "<LcCDP_CellLowFltLevel3_mV>"

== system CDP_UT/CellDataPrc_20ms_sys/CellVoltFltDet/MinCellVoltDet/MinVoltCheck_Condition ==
  GbCDP_SumCellVoltVld_flg : Inport
  GeMSM_BMUState_enum : Inport  Port=2
  LbCDP_AnyCellVoltVld_flg : Inport  Port=3
  Constant : Constant  Value=ASWTYPE_TRUE
  Constant1 : Constant  Value=CbCDP_MinCellVoltStateCheck_flg
  Constant2 : Constant  Value=ASWTYPE_TRUE
  Constant3 : Constant  Value=Enum_MSMBMUState.Enum_MSMBMUState_Run
  Constant4 : Constant  Value=ASWTYPE_TRUE
  Data Type Conversion1 : DataTypeConversion
  Logical Operator : Logic  Inputs=3  AllPortsSameDT=off  OutDataTypeStr=boolean
  Relational Operator{,1..2,4} (4 alike) : RelationalOperator  Operator===  OutDataTypeStr=boolean
  Terminator : Terminator
  LbCDP_MinVoltCheckCondition_flg : Outport
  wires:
  Logical Operator/1 -> LbCDP_MinVoltCheckCondition_flg/1  "LbCDP_MinVoltCheckCondition_flg"
  Relational Operator/1 -> Terminator/1
  Constant/1 -> Relational Operator/2
  GbCDP_SumCellVoltVld_flg/1 -> Relational Operator/1
  Relational Operator1/1 -> Logical Operator/2
  Constant2/1 -> Relational Operator1/2
  Constant1/1 -> Relational Operator1/1
  GeMSM_BMUState_enum/1 -> Data Type Conversion1/1
  Constant3/1 -> Relational Operator4/2
  Relational Operator4/1 -> Logical Operator/3
  Data Type Conversion1/1 -> Relational Operator4/1
  LbCDP_AnyCellVoltVld_flg/1 -> Relational Operator2/1
  Constant4/1 -> Relational Operator2/2
  Relational Operator2/1 -> Logical Operator/1

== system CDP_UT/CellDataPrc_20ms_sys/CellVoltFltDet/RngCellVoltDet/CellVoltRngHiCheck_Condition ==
  GbCDP_SumCellVoltVld_flg : Inport
  GeMSM_BMUState_enum : Inport  Port=2
  LbCDP_AnyCellVoltVld_flg : Inport  Port=3
  Constant : Constant  Value=ASWTYPE_TRUE
  Constant1 : Constant  Value=CbCDP_MaxCellVoltStateCheck_flg
  Constant2 : Constant  Value=ASWTYPE_TRUE
  Constant3 : Constant  Value=Enum_MSMBMUState.Enum_MSMBMUState_Run
  Constant4 : Constant  Value=ASWTYPE_TRUE
  Data Type Conversion1 : DataTypeConversion
  Logical Operator : Logic  Inputs=3  AllPortsSameDT=off  OutDataTypeStr=boolean
  Relational Operator{,1..2,4} (4 alike) : RelationalOperator  Operator===  OutDataTypeStr=boolean
  Terminator : Terminator
  LbCDP_CellVoltRngHiChk_flg : Outport
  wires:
  Logical Operator/1 -> LbCDP_CellVoltRngHiChk_flg/1  "LbCDP_CellVoltRngHiChk_flg"
  Relational Operator/1 -> Terminator/1
  Constant/1 -> Relational Operator/2
  GbCDP_SumCellVoltVld_flg/1 -> Relational Operator/1
  Relational Operator1/1 -> Logical Operator/2
  Constant2/1 -> Relational Operator1/2
  Constant1/1 -> Relational Operator1/1
  GeMSM_BMUState_enum/1 -> Data Type Conversion1/1
  Constant3/1 -> Relational Operator4/2
  Relational Operator4/1 -> Logical Operator/3
  Data Type Conversion1/1 -> Relational Operator4/1
  LbCDP_AnyCellVoltVld_flg/1 -> Relational Operator2/1
  Constant4/1 -> Relational Operator2/2
  Relational Operator2/1 -> Logical Operator/1

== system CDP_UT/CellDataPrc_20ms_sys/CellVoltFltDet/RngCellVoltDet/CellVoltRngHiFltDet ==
  LbCDP_CellVoltRngHiChk_flg : Inport
  GcCDP_MaxCellVolt_mV : Inport  Port=2
  CDP_GbCDP_ChrgMaxCellVoltFltLv1_flg : AIWAYS_Powertrain_BMS_lib/Signals/OverWrite  OverWrite_Value=CbCDP_CellVoltRngHiFltOvr_flg  OverWrite_flag=CbCDP_CellVoltRngHiFltOvrSwt_flg
  Comparison1 : RelationalOperator  OutDataTypeStr=boolean
  Constant2 : Constant  Value=CcCDP_CellVoltRngHiThrd_mV
  Constant4 : Constant  Value=ASWTYPE_TRUE
  Logical Operator : Logic  AllPortsSameDT=off  OutDataTypeStr=boolean
  Relational Operator2 : RelationalOperator  Operator===  OutDataTypeStr=boolean
  GbCDP_CellVoltRngHiFlt_flg : Outport
  LbCDP_CellVoltRngHiFlt_flg : Outport  Port=2
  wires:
  CDP_GbCDP_ChrgMaxCellVoltFltLv1_flg/1 -> GbCDP_CellVoltRngHiFlt_flg/1  "GbCDP_CellVoltRngHiFlt_flg"
  Constant2/1 -> Comparison1/2
  Comparison1/1 -> Logical Operator/1
  GcCDP_MaxCellVolt_mV/1 -> Comparison1/1
  Constant4/1 -> Relational Operator2/2
  LbCDP_CellVoltRngHiChk_flg/1 -> Relational Operator2/1
  Relational Operator2/1 -> Logical Operator/2
  Logical Operator/1 -> LbCDP_CellVoltRngHiFlt_flg/1, CDP_GbCDP_ChrgMaxCellVoltFltLv1_flg/1  "LbCDP_CellVoltRngHiFlt_flg"

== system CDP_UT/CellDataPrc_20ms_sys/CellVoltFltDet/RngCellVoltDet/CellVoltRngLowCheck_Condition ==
  GbCDP_SumCellVoltVld_flg : Inport
  GeMSM_BMUState_enum : Inport  Port=2
  LbCDP_AnyCellVoltVld_flg : Inport  Port=3
  Constant : Constant  Value=ASWTYPE_TRUE
  Constant1 : Constant  Value=CbCDP_MinCellVoltStateCheck_flg
  Constant2 : Constant  Value=ASWTYPE_TRUE
  Constant3 : Constant  Value=Enum_MSMBMUState.Enum_MSMBMUState_Run
  Constant4 : Constant  Value=ASWTYPE_TRUE
  Data Type Conversion1 : DataTypeConversion
  Logical Operator : Logic  Inputs=3  AllPortsSameDT=off  OutDataTypeStr=boolean
  Relational Operator{,1..2,4} (4 alike) : RelationalOperator  Operator===  OutDataTypeStr=boolean
  Terminator : Terminator
  LbCDP_CellVoltRngLowChk_flg : Outport
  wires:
  Data Type Conversion1/1 -> Relational Operator4/1
  Relational Operator4/1 -> Logical Operator/3
  Constant3/1 -> Relational Operator4/2
  GeMSM_BMUState_enum/1 -> Data Type Conversion1/1
  Constant1/1 -> Relational Operator1/1
  Constant2/1 -> Relational Operator1/2
  Relational Operator1/1 -> Logical Operator/2
  GbCDP_SumCellVoltVld_flg/1 -> Relational Operator/1
  Constant/1 -> Relational Operator/2
  Relational Operator/1 -> Terminator/1
  Logical Operator/1 -> LbCDP_CellVoltRngLowChk_flg/1  "LbCDP_CellVoltRngLowChk_flg"
  Constant4/1 -> Relational Operator2/2
  LbCDP_AnyCellVoltVld_flg/1 -> Relational Operator2/1
  Relational Operator2/1 -> Logical Operator/1

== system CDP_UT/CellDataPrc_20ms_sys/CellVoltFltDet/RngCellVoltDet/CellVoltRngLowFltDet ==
  LbCDP_CellVoltRngLowChk_flg : Inport
  GcCDP_MinCellVolt_mV : Inport  Port=2
  CDP_GbCDP_ChrgMaxCellVoltFltLv1_flg : AIWAYS_Powertrain_BMS_lib/Signals/OverWrite  OverWrite_Value=CbCDP_CellVoltRngLowFltOvr_flg  OverWrite_flag=CbCDP_CellVoltRngLowFltOvrSwt_flg
  Constant2 : Constant  Value=CcCDP_CellVoltRngLowThrd_mV
  Constant4 : Constant  Value=ASWTYPE_TRUE
  Logical Operator : Logic  AllPortsSameDT=off  OutDataTypeStr=boolean
  Relational Operator1 : RelationalOperator  Operator=<=  OutDataTypeStr=boolean
  Relational Operator2 : RelationalOperator  Operator===  OutDataTypeStr=boolean
  GbCDP_CellVoltRngLowFlt_flg : Outport
  LbCDP_CellVoltRngLowFlt_flg : Outport  Port=2
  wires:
  GcCDP_MinCellVolt_mV/1 -> Relational Operator1/1
  Relational Operator1/1 -> Logical Operator/1
  Constant2/1 -> Relational Operator1/2
  CDP_GbCDP_ChrgMaxCellVoltFltLv1_flg/1 -> GbCDP_CellVoltRngLowFlt_flg/1  "GbCDP_CellVoltRngLowFlt_flg"
  LbCDP_CellVoltRngLowChk_flg/1 -> Relational Operator2/1
  Constant4/1 -> Relational Operator2/2
  Relational Operator2/1 -> Logical Operator/2
  Logical Operator/1 -> LbCDP_CellVoltRngLowFlt_flg/1, CDP_GbCDP_ChrgMaxCellVoltFltLv1_flg/1  "LbCDP_CellVoltRngLowFlt_flg"

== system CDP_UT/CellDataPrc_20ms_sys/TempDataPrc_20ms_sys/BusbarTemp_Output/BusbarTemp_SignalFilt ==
  GcUDS_BusbarTempNumb_numb : Inport
  GeUDS_CapSel_enum : Inport  Port=2
  LaCDP_BusbarTempUpdateVld_flg : Inport  Port=3
  LaCDP_BusbarTemp_C : Inport  Port=4
  1D_Config_Word : AIWAYS_Powertrain_BMS_lib/Signals/1D_Config_Word  Default_CalPar_Name=CcCDP_CATL203CellTempFilCfig_numb  CATL153Ah_CalPar_Name=CcCDP_CATL177CellTempFilCfig_numb  CATL180Ah_CalPar_Name=CcCDP_CATL177CellTempFilCfig_numb  CATL177Ah_CalPar_Name=CcCDP_CATL177CellTempFilCfig_numb  CATL203Ah_CalPar_Name=CcCDP_CATL203CellTempFilCfig_numb  CATL51Ah_CalPar_Name=CcCDP_CATL177CellTempFilCfig_numb  CATL132Ah_CalPar_Name=CcCDP_CATL177CellTempFilCfig_numb  XWD75Ah_CalPar_Name=CcCDP_CATL177CellTempFilCfig_numb  TFE177Ah_CalPar_Name=CcCDP_CATL177CellTempFilCfig_numb  CATLCTP248Ah_CalPar_Name=CcCDP_CATL177CellTempFilCfig_numb
  Comparison1 : RelationalOperator  Operator===  OutDataTypeStr=boolean
  Constant6 : Constant  Value=ASWTYPE_FALSE
  InputValueCalc : Stateflow chart  TreatAsAtomicUnit=on
  MaxValue_sort : Stateflow chart  TreatAsAtomicUnit=on
  SignalDelay1 : Subsystem  Commented=on
  Terminator : Terminator
  Unit Delay21 : UnitDelay  SampleTime=-1  StateName=StateName
  GaCDP_BusbarTemp_C : Outport
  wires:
  Unit Delay21/1 -> InputValueCalc/4(Old_Value)
  LaCDP_BusbarTemp_C/1 -> InputValueCalc/1(Input_Value)
  1D_Config_Word/1 -> MaxValue_sort/2(Input_dim)
  InputValueCalc/1(Output_Value) -> Unit Delay21/1, MaxValue_sort/1(Input_Value)
  GeUDS_CapSel_enum/1 -> 1D_Config_Word/1
  LaCDP_BusbarTempUpdateVld_flg/1 -> Comparison1/1
  MaxValue_sort/1(Output_Value) -> Terminator/1
  GcUDS_BusbarTempNumb_numb/1 -> InputValueCalc/3(Input_num), MaxValue_sort/3(Input_num)
  MaxValue_sort/2(TargetOutput_Value) -> GaCDP_BusbarTemp_C/1  "GaCDP_BusbarTemp_C"
  Constant6/1 -> Comparison1/2
  Comparison1/1 -> InputValueCalc/2(Update)  "LaCDP_BusbarTempUpdateVld_flg"

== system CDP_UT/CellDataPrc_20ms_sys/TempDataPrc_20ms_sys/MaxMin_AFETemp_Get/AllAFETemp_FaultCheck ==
  LaCDP_AFETempVld_flg : Inport
  AFETempVld : Subsystem
  Constant4 : Constant  Value=CcCDP_AFETempConfig_numb
  LbCDP_AnyAFETempVld_flg : Outport
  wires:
  AFETempVld/1(LbCDP_AnyAFETempVld_flg) -> LbCDP_AnyAFETempVld_flg/1
  Constant4/1 -> AFETempVld/2(CcCDP_AFETempConfig_numb)
  LaCDP_AFETempVld_flg/1 -> AFETempVld/1(LaCDP_AFETempVld_flg)

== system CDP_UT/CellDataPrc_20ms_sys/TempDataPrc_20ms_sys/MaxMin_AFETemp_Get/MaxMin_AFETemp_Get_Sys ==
  LaCDP_AFETempVld_flg : Inport
  LaCDP_AFETemp_C : Inport  Port=2
  Enable : EnablePort  StatesWhenEnabling=reset
  CDP_GcCDP_MaxCMUPCBTempNumb_numb : AIWAYS_Powertrain_BMS_lib/Signals/OverWrite  OverWrite_Value=CcCDP_MaxAFETempNumbOvr_numb  OverWrite_flag=CbCDP_MaxAFETempNumbOvrSwt_flg
  CDP_GcCDP_MaxCMUPCBTemp_C : AIWAYS_Powertrain_BMS_lib/Signals/OverWrite  OverWrite_Value=CcCDP_MaxAFETempOvr_C  OverWrite_flag=CbCDP_MaxAFETempOvrSwt_flg
  CDP_GcCDP_MinCMUPCBTempNumb_numb : AIWAYS_Powertrain_BMS_lib/Signals/OverWrite  OverWrite_Value=CcCDP_MinAFETempNumbOvr_numb  OverWrite_flag=CbCDP_MinAFETempNumbOvrSwt_flg
  CDP_GcCDP_MinCMUPCBTemp_C : AIWAYS_Powertrain_BMS_lib/Signals/OverWrite  OverWrite_Value=CcCDP_MinAFETempOvr_C  OverWrite_flag=CbCDP_MinAFETempOvrSwt_flg
  Constant3 : Constant  Value=CcCDP_AFETempConfig_numb
  MinAFETemp_ForIterator : Subsystem  TreatAsAtomicUnit=on
  GcCDP_MaxAFETemp_C : Outport
  GcCDP_MaxAFETempNumb_numb : Outport  Port=2
  GcCDP_MinAFETemp_C : Outport  Port=3
  GcCDP_MinAFETempNumb_numb : Outport  Port=4
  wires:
  MinAFETemp_ForIterator/4(LcCDP_MaxAFETemp_C) -> CDP_GcCDP_MaxCMUPCBTemp_C/1
  MinAFETemp_ForIterator/3(LcCDP_MaxAFETempNumb_numb) -> CDP_GcCDP_MaxCMUPCBTempNumb_numb/1
  CDP_GcCDP_MaxCMUPCBTemp_C/1 -> GcCDP_MaxAFETemp_C/1  "GcCDP_MaxAFETemp_C"
  CDP_GcCDP_MaxCMUPCBTempNumb_numb/1 -> GcCDP_MaxAFETempNumb_numb/1  "GcCDP_MaxAFETempNumb_numb"
  CDP_GcCDP_MinCMUPCBTemp_C/1 -> GcCDP_MinAFETemp_C/1  "GcCDP_MinAFETemp_C"
  CDP_GcCDP_MinCMUPCBTempNumb_numb/1 -> GcCDP_MinAFETempNumb_numb/1  "GcCDP_MinAFETempNumb_numb"
  LaCDP_AFETempVld_flg/1 -> MinAFETemp_ForIterator/2(LaCDP_AFETempVld_flg)
  MinAFETemp_ForIterator/2(LcCDP_MinAFETempNumb_numb) -> CDP_GcCDP_MinCMUPCBTempNumb_numb/1
  MinAFETemp_ForIterator/1(LcCDP_MinAFETemp_C) -> CDP_GcCDP_MinCMUPCBTemp_C/1
  LaCDP_AFETemp_C/1 -> MinAFETemp_ForIterator/1(LaCDP_AFETemp_C)
  Constant3/1 -> MinAFETemp_ForIterator/3(CcCDP_AFETempConfig_numb)

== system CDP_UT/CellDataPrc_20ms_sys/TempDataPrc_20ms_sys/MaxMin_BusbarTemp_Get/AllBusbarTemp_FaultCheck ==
  LaCDP_BusbarTempVld_flg : Inport
  GcUDS_BusbarTempNumb_numb : Inport  Port=2
  GaISP_BusbarTempUpdCnt_numb : Inport  Port=3
  BusbarTempVld : Subsystem
  Comparison4 : RelationalOperator  Operator===  OutDataTypeStr=boolean
  Constant1 : Constant  Value=CDP_CONST0_NUMB
  Constant2 : Constant  Value=CbCDP_IgnorUpdateVld_flg
  Logical : Logic  OutDataTypeStr=boolean
  OverWrite : AIWAYS_Powertrain_BMS_lib/Signals/OverWrite  OverWrite_Value=CbCDP_AllBusbarTempVldOvr_flg  OverWrite_flag=CbCDP_AllBusbarTempVldOvrSwt_flg
  Switch : Switch  Criteria=u2 ~= 0  Threshold=1  RndMeth=Zero
  GbCDP_AllBusbarTempVld_flg : Outport
  LbCDP_AnyBusbarTempVld_flg : Outport  Port=2
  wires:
  BusbarTempVld/2(LbCDP_AnyBusbarTempVld_flg) -> LbCDP_AnyBusbarTempVld_flg/1
  GcUDS_BusbarTempNumb_numb/1 -> BusbarTempVld/2(GcUDS_BusbarTempNumb_numb)
  OverWrite/1 -> GbCDP_AllBusbarTempVld_flg/1  "GbCDP_AllBusbarTempVld_flg"
  BusbarTempVld/1(LbCDP_BusbarTempVld_flg) -> OverWrite/1
  GaISP_BusbarTempUpdCnt_numb/1 -> Comparison4/1
  Comparison4/1 -> Logical/2
  Constant1/1 -> Comparison4/2
  LaCDP_BusbarTempVld_flg/1 -> Switch/1, Logical/1
  Logical/1 -> Switch/3
  Constant2/1 -> Switch/2
  Switch/1 -> BusbarTempVld/1(LaCDP_BusbarTempVld_flg)

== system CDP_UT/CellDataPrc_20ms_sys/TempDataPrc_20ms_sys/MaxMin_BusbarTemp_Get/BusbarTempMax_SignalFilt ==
  LcCDP_MaxBusbarTemp_C : Inport
  LcCDP_MaxBusbarTempNumb_numb : Inport  Port=2
  LbCDP_AnyBusbarTempVld_flg : Inport  Port=3
  GeUDS_CapSel_enum : Inport  Port=4
  1D_Config_Word : AIWAYS_Powertrain_BMS_lib/Signals/1D_Config_Word  Default_CalPar_Name=CcCDP_CATL203MaxCellTempFilCfig_numb  CATL153Ah_CalPar_Name=CcCDP_CATL177MaxCellTempFilCfig_numb  CATL180Ah_CalPar_Name=CcCDP_CATL177MaxCellTempFilCfig_numb  CATL177Ah_CalPar_Name=CcCDP_CATL177MaxCellTempFilCfig_numb  CATL203Ah_CalPar_Name=CcCDP_CATL203MaxCellTempFilCfig_numb  CATL51Ah_CalPar_Name=CcCDP_CATL177MaxCellTempFilCfig_numb  CATL132Ah_CalPar_Name=CcCDP_CATL177MaxCellTempFilCfig_numb  XWD75Ah_CalPar_Name=CcCDP_CATL177MaxCellTempFilCfig_numb  TFE177Ah_CalPar_Name=CcCDP_CATL177MaxCellTempFilCfig_numb  CATLCTP248Ah_CalPar_Name=CcCDP_CATL177MaxCellTempFilCfig_numb
  InputValueCalc : Stateflow chart  TreatAsAtomicUnit=on
  MaxValue_sort : Stateflow chart  TreatAsAtomicUnit=on
  SignalDelay1 : Subsystem  Commented=on
  Unit Delay21 : UnitDelay  SampleTime=-1  StateName=StateName
  ValueCalc : Subsystem
  ValueIndexCalc : Subsystem
  GcCDP_MaxBusbarTemp_C : Outport
  GcCDP_MaxBusbarTempNumb_numb : Outport  Port=2
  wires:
  ValueCalc/2(Output_index1) -> ValueIndexCalc/1(Output_index1)
  MaxValue_sort/2(Output_index) -> ValueCalc/2(Output_index)
  MaxValue_sort/1(Output_Value) -> ValueCalc/1(Output_Value)
  Unit Delay21/1 -> InputValueCalc/3(Old_Value)
  LcCDP_MaxBusbarTemp_C/1 -> InputValueCalc/1(Input_Value)
  LcCDP_MaxBusbarTempNumb_numb/1 -> ValueIndexCalc/2(LcCDP_MaxBusbarTempNumb_numb)
  ValueIndexCalc/1(GcCDP_MaxBusbarTempNumb_numb) -> GcCDP_MaxBusbarTempNumb_numb/1
  ValueCalc/1(GcCDP_MaxBusbarTemp_C) -> GcCDP_MaxBusbarTemp_C/1
  1D_Config_Word/1 -> MaxValue_sort/2(Input_dim), ValueCalc/3(CcCDP_CellTempFilConfig_numb)
  InputValueCalc/1(Output_Value) -> MaxValue_sort/1(Input_Value), Unit Delay21/1
  GeUDS_CapSel_enum/1 -> 1D_Config_Word/1
  LbCDP_AnyBusbarTempVld_flg/1 -> ValueIndexCalc/3(LbCDP_AnyBusbarTempVld_flg), InputValueCalc/2(Rige)
